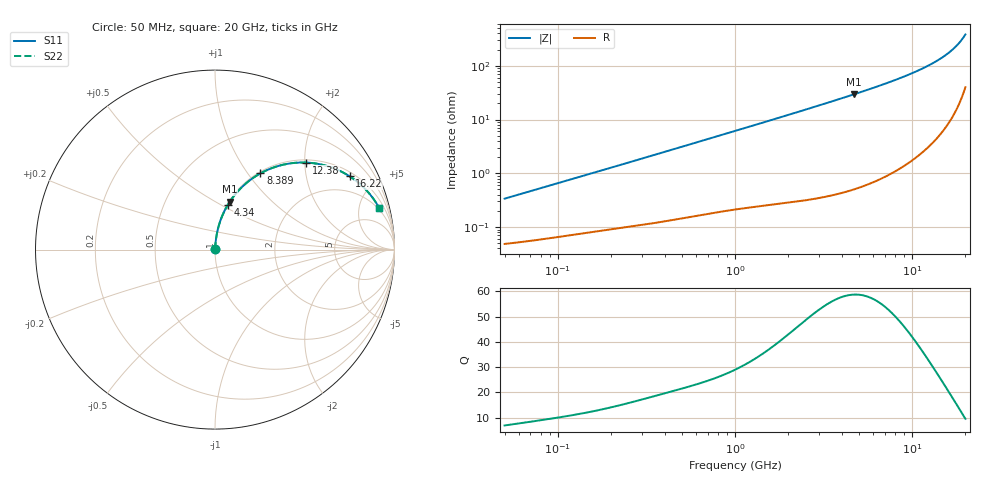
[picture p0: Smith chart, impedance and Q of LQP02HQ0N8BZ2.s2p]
!Murata Part Number: LQP02HQ0N8BZ2
!These Parameters are Measured in Series Mode Connection
!  o--[Z]--o
!Port1  Port2
!  o-------o
!Freq. Start=50[MHz] Stop=20[GHz], 401[Steps]
# Hz S RI R 50
!Freq.(Hz) S11(Real) S11(Imag) S21(Real) S21(Imag) S12(Real) S12(Imag) S22(Real) S22(Imag)
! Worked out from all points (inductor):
!   401 points, 50 MHz to 20 GHz, reference 50 ohm
!   read as one part in series: L = 1.05 nH near 51.52 MHz
!   highest Q = 58.7 at 4.678 GHz (marker M1), where L = 998 pH
!   S11 on the Smith chart (normalised r, x): 50 MHz: 1.00, +0.01; 4.34 GHz: 1.01, +0.54; 8.389 GHz: 1.02, +1.15; 12.38 GHz: 1.06, +2.03; 16.22 GHz: 1.18, +3.56; 20 GHz: 1.80, +7.62
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5e7  0.000496 0.00334  0.9995 -0.00334  0.9995 -0.00334  0.000496 0.00334
1.364002e8  0.000833 0.00878  0.9992 -0.00878  0.9992 -0.00878  0.000833 0.00878
3.721004e8  0.00176 0.0232  0.9982 -0.0232  0.9982 -0.0232  0.00176 0.0232
1e9  0.00583 0.0608  0.9942 -0.0608  0.9942 -0.0608  0.00583 0.0608
1.714689e9  0.0134 0.1029  0.9866 -0.1029  0.9866 -0.1029  0.0134 0.1029
2.728004e9  0.0302 0.1616  0.9698 -0.1616  0.9698 -0.1616  0.0302 0.1616
4.34015e9  0.072 0.2501  0.928 -0.2501  0.928 -0.2501  0.072 0.2501
4.677679e9  0.0831 0.2677  0.9169 -0.2677  0.9169 -0.2677  0.0831 0.2677
6.034176e9  0.1354 0.3335  0.8646 -0.3335  0.8646 -0.3335  0.1354 0.3335
7.442007e9  0.2021 0.3921  0.7979 -0.3921  0.7979 -0.3921  0.2021 0.3921
8.389408e9  0.2533 0.4248  0.7467 -0.4248  0.7467 -0.4248  0.2533 0.4248
1.019291e10  0.3622 0.4687  0.6378 -0.4687  0.6378 -0.4687  0.3622 0.4687
1.131968e10  0.4355 0.4824  0.5645 -0.4824  0.5645 -0.4824  0.4355 0.4824
1.238412e10  0.5066 0.4849  0.4934 -0.4849  0.4934 -0.4849  0.5066 0.4849
1.417136e10  0.6251 0.4655  0.3749 -0.4655  0.3749 -0.4655  0.6251 0.4655
1.527346e10  0.6944 0.4392  0.3056 -0.4392  0.3056 -0.4392  0.6944 0.4392
1.621653e10  0.7497 0.4088  0.2503 -0.4088  0.2503 -0.4088  0.7497 0.4088
1.721783e10  0.803 0.3693  0.197 -0.3693  0.197 -0.3693  0.803 0.3693
1.800918e10  0.8406 0.3336  0.1594 -0.3336  0.1594 -0.3336  0.8406 0.3336
1.88369e10  0.8752 0.2929  0.1248 -0.2929  0.1248 -0.2929  0.8752 0.2929
1.940974e10  0.8961 0.2631  0.1039 -0.2631  0.1039 -0.2631  0.8961 0.2631
2e10  0.915 0.2312  0.085 -0.2312  0.085 -0.2312  0.915 0.2312
